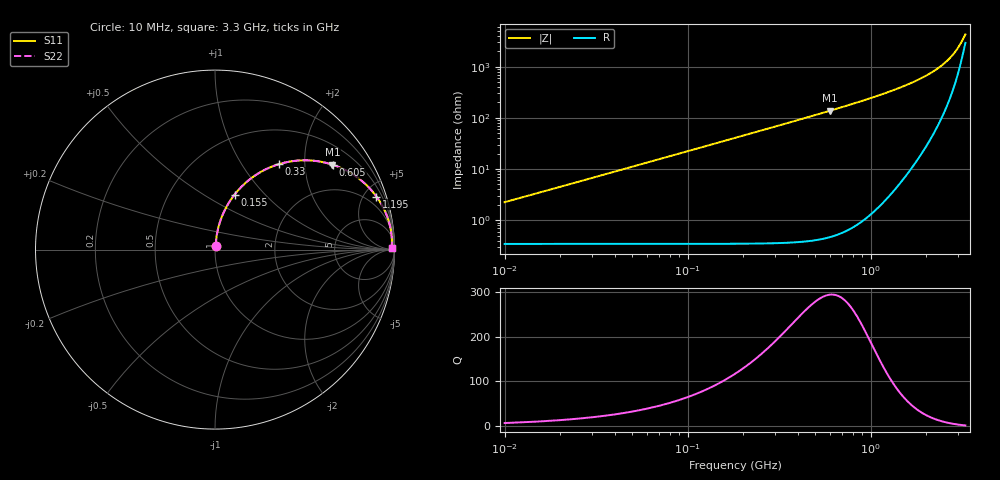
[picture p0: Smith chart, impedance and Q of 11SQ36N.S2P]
! Coilcraft 1111SQ-36N Air Core Inductor
! 14 MAR 2012
# MHZ S MA R 50
!Freq  MagS11  AngS11  MagS21  AngS21  MagS12  AngS12  MagS22  AngS22
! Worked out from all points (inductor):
!   659 points, 10 MHz to 3.3 GHz, reference 50 ohm
!   read as one part in series: L = 35.5 nH near 25 MHz
!   highest Q = 294 at 600 MHz (marker M1), where L = 36.5 nH
!   S11 on the Smith chart (normalised r, x): 10 MHz: 1.01, +0.04; 155 MHz: 1.01, +0.69; 330 MHz: 1.01, +1.48; 605 MHz: 1.01, +2.78; 1.195 GHz: 1.07, +6.07; 3.3 GHz: open
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10  0.02245 79.9  0.9963 -1.3  0.9963 -1.3  0.02245 79.9
20  0.04447 83.0  0.9956 -2.5  0.9956 -2.5  0.04447 83.0
35  0.07751 83.0  0.9936 -4.4  0.9936 -4.4  0.07751 83.0
45  0.09942 82.3  0.9916 -5.7  0.9916 -5.7  0.09942 82.3
60  0.132 80.9  0.9878 -7.6  0.9878 -7.6  0.132 80.9
80  0.1749 78.8  0.9812 -10.1  0.9812 -10.1  0.1749 78.8
100  0.2168 76.6  0.9729 -12.5  0.9729 -12.5  0.2168 76.6
155  0.3258 70.4  0.9422 -19.0  0.9422 -19.0  0.3258 70.4
230  0.4561 62.4  0.8868 -27.2  0.8868 -27.2  0.4561 62.4
330  0.5941 53.2  0.8015 -36.5  0.8015 -36.5  0.5941 53.2
430  0.6956 45.6  0.7157 -44.1  0.7157 -44.1  0.6956 45.6
560  0.7866 37.9  0.6147 -51.9  0.6147 -51.9  0.7866 37.9
600  0.8077 35.9  0.5869 -54.0  0.5869 -54.0  0.8077 35.9
605  0.8101 35.6  0.5835 -54.2  0.5835 -54.2  0.8102 35.6
830  0.8891 26.9  0.4541 -62.9  0.4541 -62.9  0.8891 26.9
1110  0.9377 19.8  0.3413 -69.8  0.3413 -69.8  0.9377 19.8
1195  0.9468 18.2  0.3144 -71.4  0.3144 -71.4  0.9468 18.2
1655  0.9744 11.6  0.2056 -77.2  0.2056 -77.2  0.9744 11.6
2205  0.9853 6.7  0.1218 -79.9  0.1218 -79.9  0.9853 6.7
2755  0.9869 3.2  0.06333 -76.6  0.06333 -76.6  0.9869 3.2
3010  0.9859 1.9  0.04196 -69.7  0.04196 -69.7  0.9859 1.9
3300  0.984 0.5  0.02314 -46.3  0.02314 -46.3  0.984 0.5
